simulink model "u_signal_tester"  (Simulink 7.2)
settings: Solver=ode23tb  StartTime=0.0  StopTime=1000  MaxStep=.1  RelTol=1e-3
undefined symbols (not defined in the file or in its folder): sigbuilder_block

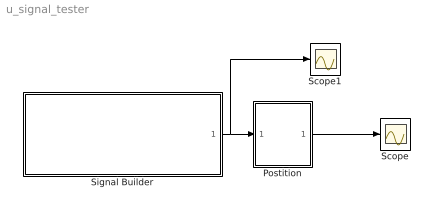
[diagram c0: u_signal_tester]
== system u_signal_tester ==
  Postition : Subsystem
  Scope : Scope
  Scope1 : Scope
  Signal Builder : Subsystem  Tag=STV Subsys  LoadFcn=sigbuilder_block('load');  StartFcn=sigbuilder_block('start');  StopFcn=sigbuilder_block('stop');  ClipboardFcn=sigbuilder_block('clipboard');
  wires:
  Postition/1(x) -> Scope/1
  Signal Builder/1(u) -> Postition/1(u), Scope1/1

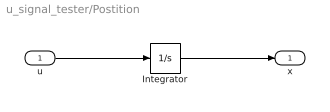
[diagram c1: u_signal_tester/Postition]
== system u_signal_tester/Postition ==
  u : Inport  OutDataType=sfix(16)  OutScaling=2^0
  Integrator : Integrator  LimitOutput=on  UpperSaturationLimit=1  LowerSaturationLimit=0
  x : Outport  OutDataType=sfix(16)  OutScaling=2^0
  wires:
  u/1 -> Integrator/1
  Integrator/1 -> x/1

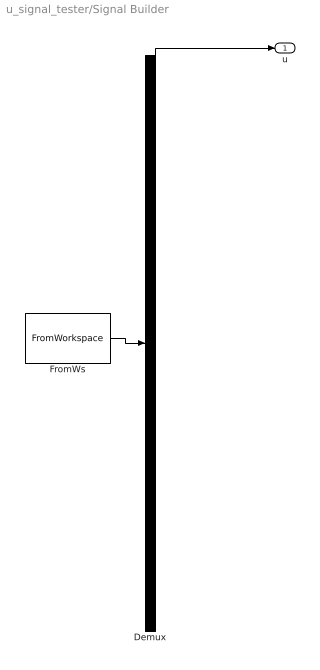
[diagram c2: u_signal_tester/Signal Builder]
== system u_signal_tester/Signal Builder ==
  Demux : Demux  Tag=STV Demux  Outputs=1
  FromWs : FromWorkspace  Tag=STV FromWs  VariableName=tuvar  SampleTime=0  SigBuilderData=DataTag0  VnvData=DataTag1
  u : Outport  Tag=STV Outport
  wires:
  FromWs/1 -> Demux/1
  Demux/1 -> u/1
